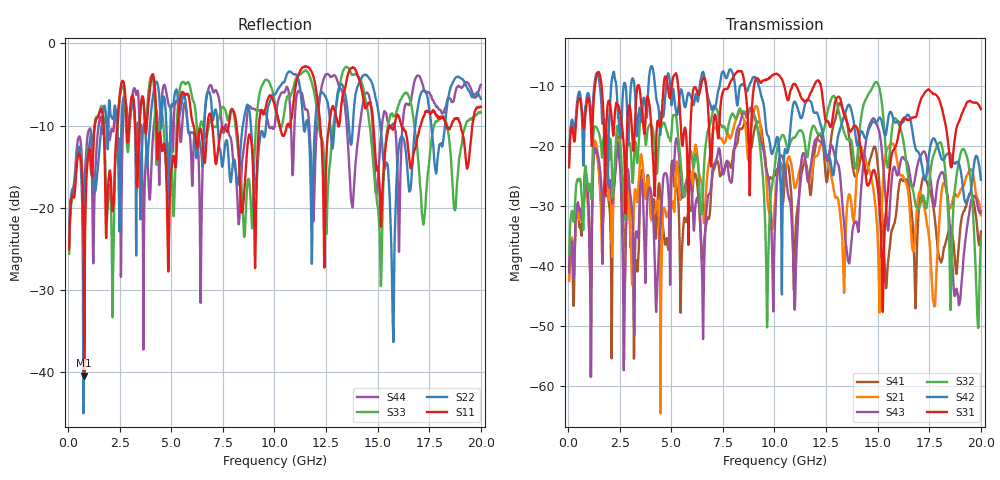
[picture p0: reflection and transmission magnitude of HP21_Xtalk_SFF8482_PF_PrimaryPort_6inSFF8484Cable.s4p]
# MHz S MA R 50.00
! FREQ  S11  S12  S13  S14
!  S21  S22  S23  S24
!  S31  S32  S33  S34
!  S41  S42  S43  S44
!  MAG  ANG  MAG  ANG  MAG  ANG  MAG  ANG
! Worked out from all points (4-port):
!   1996 points, 50 MHz to 20 GHz, reference 50 ohm
!   strongest paths, dB at 50 MHz, 5.04 GHz, 10.03 GHz, 15.02 GHz, 20 GHz:
!     S31: -23.5, -9.4, -8.0, -27.4, -13.8
!     S42: -22.5, -12.1, -19.9, -15.6, -25.6
!     S32: -38.1, -16.1, -22.9, -9.7, -35.9
!     S43: -41.0, -22.8, -32.5, -16.9, -30.9
!     S21: -42.5, -29.9, -29.0, -37.3, -31.5
!     S41: -42.2, -22.5, -24.9, -23.8, -34.3
!   lowest |S11| = -40.4 dB at 780 MHz (marker M1), VSWR 1.02, Z = 49.7 + j0.89 ohm
!   |S11| at or under -10 dB: start of sweep to 1.3 GHz; 4.288 GHz to 5.315 GHz (1.027 GHz wide, 21.4 % of centre); 8.162 GHz to 9.247 GHz (1.085 GHz wide, 12.5 % of centre)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
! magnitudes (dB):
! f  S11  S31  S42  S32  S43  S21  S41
! 50 MHz  -25.0  -23.5  -22.5  -38.1  -41.0  -42.5  -42.2
! 780 MHz  -40.4  -17.1  -18.3  -28.7  -28.5  -27.1  -28.1
! 6.53 GHz  -12.5  -8.7  -7.6  -28.0  -50.6  -29.5  -38.5
! 8.79 GHz  -11.1  -27.1  -9.8  -14.0  -13.9  -20.1  -19.5
! 9.65 GHz  -7.0  -8.9  -18.1  -49.1  -24.5  -28.3  -25.4
! 14.93 GHz  -15.1  -25.3  -16.0  -9.3  -16.2  -31.5  -20.9
! 20 GHz  -7.7  -13.8  -25.6  -35.9  -30.9  -31.5  -34.3
